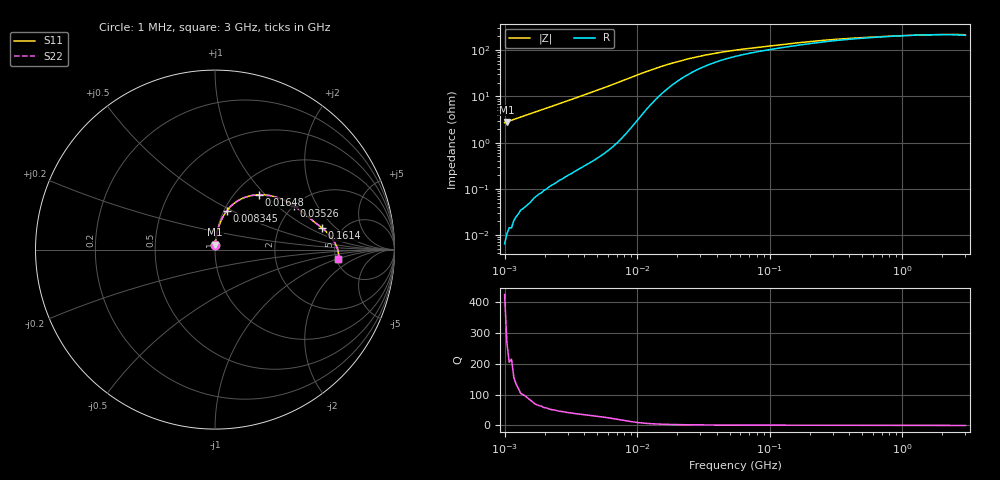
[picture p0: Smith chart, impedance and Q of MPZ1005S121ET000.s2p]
! S-Parameter Data Generated by TDK Corporation
! Copyright(C) 2025 TDK Corporation.
! All Rights Reserved.
! TDK P/N: MPZ1005S121ET000 (Chip Bead)
! Property: |Z|=120ohm at 100MHz
! Size(LxWxT): 1x0.5x0.5mm
! Model Type: s2p (Touchstone File Format Version 1.0)
! Frequency: DC=Yes Start=1MHz Stop=3000MHz 202points Log-sweep
! Model Generated on Feb. 6, 2025
! Terms and conditions regarding TDK Simulation Models:
! 1)This simulation model is being provided solely for informational
!  purposes. Please refer to the specifications of the products in
!  terms of detailed characteristics of such products.
! 2)In no event shall TDK Corporation of any of its subsidiaries be
!  liable for any loss or damage arising, directly or indirectly,
!  from any information contained in this simulation model, including,
!  but not limited to loss or damages arising from any inaccuracies,
!  omissions or errors in connection with such information.
! 3)Any and all copyrights on this simulation model are owned by
!  TDK Corporation.  Duplication or redistribution of this simulation
!  model without prior written permission from TDK Corporation
!  is prohibited.
! 4)This simulation model is subject to any modification or change
!  without any prior notice.
! 5)Neither TDK Corporation nor any of its subsidiaries shall make any
!  warranty, express or implied, including but not limited to the
!  correctness, implied warranties of merchantability and fitness for
!  a particular purpose with respect to this simulation models.
! 6)The use of this simulation model shall be deemed to have consented
!  to the terms and conditions hereof.
! Port Assignments:
!  1 ---@@@--- 2
! Applicable Conditions:
!  Temperature = 25 degC
!  DC Bias Current = 0 A
!  Small Signal Operation
# Hz S MA R 50
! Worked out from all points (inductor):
!   201 points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, 1 MHz to 3 GHz, reference 50 ohm
!   read as one part in series: L = 431 nH near 1.041 MHz
!   highest Q = 268 at 1.041 MHz (marker M1), where L = 431 nH
!   self-resonance near 1.479 GHz
!   S11 on the Smith chart (normalised r, x): 1 MHz: 1.00, +0.05; 8.345 MHz: 1.03, +0.47; 16.48 MHz: 1.28, +0.92; 35.26 MHz: 2.00, +1.31; 161.4 MHz: 3.56, +1.36; 3 GHz: 5.21, -0.99
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1000000  0.0271 88.3  0.9996 -1.6  0.9996 -1.6  0.0271 88.3
1040844  0.02816 88.2  0.9995 -1.6  0.9995 -1.6  0.02816 88.2
2226959  0.05984 85.5  0.9971 -3.4  0.9971 -3.4  0.05984 85.5
3900413  0.1046 82.4  0.9916 -6.0  0.9916 -6.0  0.1046 82.4
6058321  0.1634 78.3  0.9799 -9.4  0.9799 -9.4  0.1634 78.3
8345207  0.2277 72.9  0.9582 -13.1  0.9582 -13.1  0.2277 72.9
1.104425e7  0.2975 65.3  0.9164 -17.2  0.9164 -17.2  0.2975 65.3
1.29622e7  0.3378 59.9  0.8803 -19.4  0.8803 -19.4  0.3378 59.9
1.461624e7  0.3658 55.6  0.8488 -20.8  0.8488 -20.8  0.3658 55.6
1.648134e7  0.3914 51.3  0.8149 -22.0  0.8149 -22.0  0.3914 51.3
2.013356e7  0.4295 44.4  0.7557 -23.4  0.7557 -23.4  0.4295 44.4
2.459509e7  0.4607 38.2  0.6989 -24.1  0.6989 -24.1  0.4607 38.2
3.526298e7  0.5026 29.1  0.612 -23.6  0.612 -23.6  0.5026 29.1
5.477226e7  0.539 21.4  0.5358 -21.6  0.5358 -21.6  0.539 21.4
8.854986e7  0.5713 16.0  0.4774 -19.2  0.4774 -19.2  0.5713 16.0
1.614254e8  0.6094 11.4  0.4201 -16.6  0.4201 -16.6  0.6094 11.4
2.136344e8  0.625 9.5  0.3972 -15.1  0.3972 -15.1  0.625 9.5
3.741707e8  0.6489 6.3  0.362 -11.3  0.362 -11.3  0.6489 6.3
8.005644e8  0.6709 2.8  0.3316 -5.7  0.3316 -5.7  0.6709 2.8
1.855641e9  0.6869 -1.2  0.3136 2.5  0.3136 2.5  0.6869 -1.2
2.455801e9  0.6897 -2.8  0.3129 6.1  0.3129 6.1  0.6897 -2.8
3e9  0.6879 -4.2  0.3178 9.0  0.3178 9.0  0.6879 -4.2
